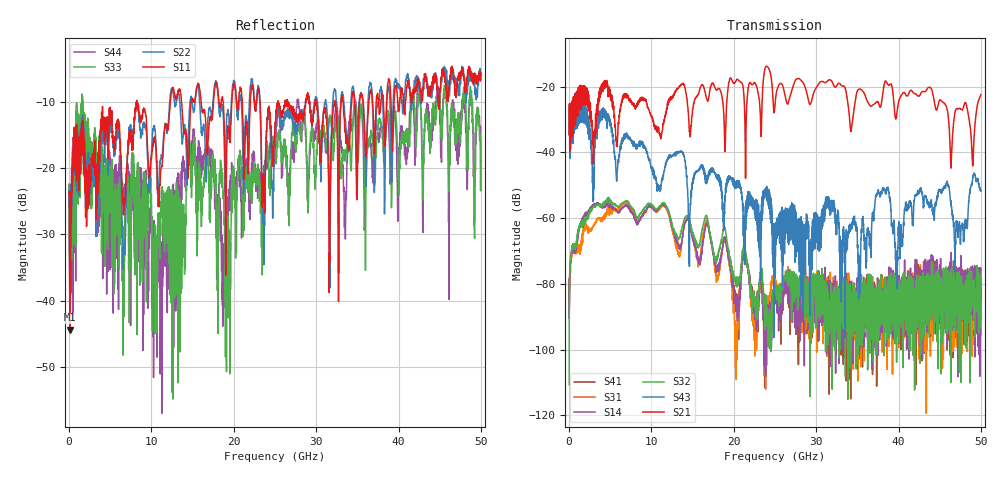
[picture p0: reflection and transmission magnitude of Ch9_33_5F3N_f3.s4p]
!Agilent Technologies,N5247A,US51170199,A.09.90.13
!Agilent N5247A: A.09.90.13
!Date: Wednesday, December 16, 2015 12:10:44
!Correction: S11(Full 4 Port(1,2,3,4))
!S12(Full 4 Port(1,2,3,4))
!S13(Full 4 Port(1,2,3,4))
!S14(Full 4 Port(1,2,3,4))
!S21(Full 4 Port(1,2,3,4))
!S22(Full 4 Port(1,2,3,4))
!S23(Full 4 Port(1,2,3,4))
!S24(Full 4 Port(1,2,3,4))
!S31(Full 4 Port(1,2,3,4))
!S32(Full 4 Port(1,2,3,4))
!S33(Full 4 Port(1,2,3,4))
!S34(Full 4 Port(1,2,3,4))
!S41(Full 4 Port(1,2,3,4))
!S42(Full 4 Port(1,2,3,4))
!S43(Full 4 Port(1,2,3,4))
!S44(Full 4 Port(1,2,3,4))
!S4P File: Measurements: <S11,S12,S13,S14>,
!<S21,S22,S23,S24>,
!<S31,S32,S33,S34>,
!<S41,S42,S43,S44>:
# Hz S  dB  R 50
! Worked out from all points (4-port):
!   3201 points, 10 MHz to 50 GHz, reference 50 ohm
!   strongest paths, dB at 10 MHz, 12.51 GHz, 25 GHz, 37.5 GHz, 50 GHz:
!     S21: -34.4, -23.5, -25.7, -24.6, -22.4
!     S43: -34.7, -41.2, -61.7, -52.0, -51.8
!     S32: -110.7, -62.0, -80.7, -91.0, -79.9
!     S14: -84.9, -62.6, -83.6, -78.7, -75.3
!     S31: -85.7, -63.5, -79.4, -89.4, -95.3
!     S41: -78.5, -62.6, -82.6, -84.0, -84.1
!   lowest |S11| = -44.4 dB at 88.11 MHz (marker M1), VSWR 1.01, Z = 50.4 + j0.488 ohm
!   |S11| at or under -10 dB: start of sweep to 8.214 GHz; 8.25 GHz to 12.28 GHz (4.029 GHz wide, 39.3 % of centre); 23.19 GHz to 25.35 GHz (2.169 GHz wide, 8.94 % of centre)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
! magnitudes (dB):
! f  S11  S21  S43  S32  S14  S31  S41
! 10 MHz  -23.7  -34.4  -34.7  -110.7  -84.9  -85.7  -78.5
! 88.11 MHz  -44.4  -39.6  -41.8  -76.7  -77.6  -79.4  -76.7
! 6.915 GHz  -22.1  -22.6  -35.1  -54.8  -56.1  -55.4  -56.2
! 18.76 GHz  -10.6  -27.1  -63.9  -63.3  -67.1  -66.7  -67.0
! 35.24 GHz  -10.7  -20.7  -79.8  -86.6  -89.6  -85.5  -90.3
! 38.11 GHz  -8.9  -21.6  -50.9  -83.1  -93.3  -80.9  -83.5
! 50 GHz  -5.7  -22.4  -51.8  -79.9  -75.3  -95.3  -84.1
